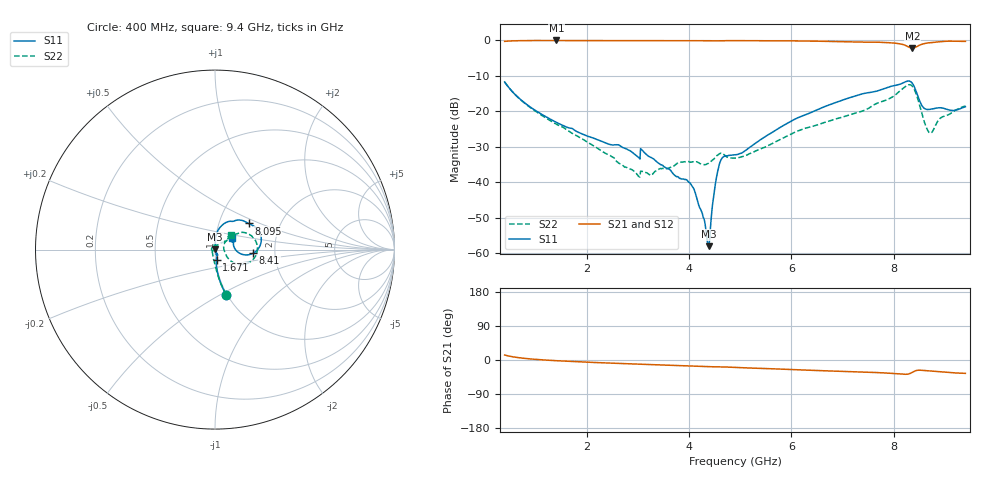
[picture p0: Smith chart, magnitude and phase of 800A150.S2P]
!  American Technical Ceramics  Date:  12/17/08
!  One Norden Lane
!  Huntington Station,  NY.  11746-2102
!  Tel:  (631) 622-4700  Fax:  (631) 622-4748
!  Part Number  800A150
!  Description: Broardband capacitor  Mounting Orientation: Vertical
!  Application:
# GHZ S DB R 50
! Freq  |S11|  S11 Ph  |S21|  S21 Ph  |S12|  S12 Ph  |S22|  S22 Ph
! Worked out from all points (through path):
!   801 points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, 400 MHz to 9.4 GHz, reference 50 ohm
!   highest |S21| = -0.07 dB at 1.413 GHz (marker M1); lowest = -2.3 dB at 8.365 GHz (marker M2)
!   group delay of S21, straight-line fit = 12.8 ps
!   lowest |S11| = -58.0 dB at 4.383 GHz (marker M3), VSWR 1.00, Z = 50.1 + j0.11 ohm
!   |S11| at or under -10 dB: start of sweep to end of sweep
!   |S22| runs from -38.5 to -11.8 dB; largest |S21 - S12| = 0.0028
!   S11 on the Smith chart (normalised r, x): 400 MHz: 0.99, -0.53; 1.671 GHz: 1.01, -0.12; 8.095 GHz: 1.38, +0.43; 8.41 GHz: 1.54, -0.06; 9.4 GHz: 1.20, +0.16
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0.4  -11.75 -76.2  -0.33 13.3  -0.33 13.3  -11.76 -76.0
1.413  -23.13 -83.9  -0.07 -1.8  -0.06 -1.9  -23.65 -93.5
1.671  -24.71 -80.4  -0.08 -3.6  -0.07 -3.7  -25.77 -99.7
1.908  -26.34 -78.8  -0.08 -5.1  -0.07 -5.1  -27.69 -104.7
2.999  -32.75 -62.5  -0.14 -10.8  -0.14 -10.8  -37.97 178.9
3.1  -31.14 -74.9  -0.13 -11.2  -0.12 -11.2  -36.99 -155.4
3.404  -34.57 -67.7  -0.09 -12.7  -0.09 -12.8  -36.40 -153.5
4.056  -40.88 -44.4  -0.13 -15.9  -0.12 -15.9  -34.25 159.9
4.383  -57.95 60.2  -0.14 -17.5  -0.14 -17.6  -34.62 137.3
4.506  -41.35 125.1  -0.19 -18.0  -0.18 -18.1  -33.13 127.2
4.596  -34.82 109.4  -0.20 -18.1  -0.19 -18.1  -31.97 112.3
4.686  -32.69 87.2  -0.15 -18.3  -0.15 -18.4  -32.21 93.9
4.9  -32.24 75.5  -0.11 -19.6  -0.10 -19.6  -33.18 78.9
6.408  -20.20 82.9  -0.26 -27.2  -0.26 -27.3  -24.27 41.6
7.904  -13.16 48.1  -0.70 -34.8  -0.71 -34.8  -16.53 36.0
8.095  -12.50 37.9  -0.95 -36.5  -0.96 -36.6  -14.60 30.9
8.365  -12.16 2.9  -2.25 -32.5  -2.25 -32.6  -12.96 -11.4
8.41  -13.38 -5.2  -2.11 -29.3  -2.11 -29.4  -14.08 -22.5
8.556  -18.52 -2.8  -1.11 -27.3  -1.11 -27.3  -20.96 -33.9
8.714  -19.43 16.2  -0.70 -29.1  -0.70 -29.2  -26.14 7.1
8.916  -19.00 21.8  -0.42 -30.8  -0.43 -30.9  -21.88 37.2
9.4  -18.71 35.4  -0.33 -35.2  -0.34 -35.3  -18.55 42.0
